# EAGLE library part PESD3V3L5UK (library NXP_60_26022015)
Low capacitance unidirectional fivefold ESD protection diode arrays Low capacitance unidirectional fivefold ElectroStatic Discharge (ESD) protection diode arrays in a leadless ultra small SOT891 Surface-Mounted Device (SMD) plastic package designed to protect up to five unidirectional signal lines from the damage caused by ESD and other transients. AAL Eindhoven MK
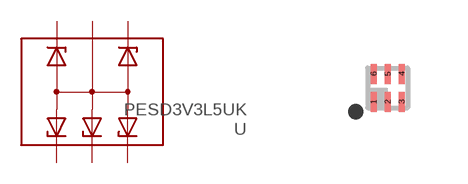
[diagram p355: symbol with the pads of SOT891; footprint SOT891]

Designator prefix U

## PESD3V3L5UK  [SOT891]
1  K1  pas
2  CA  pas
3  K2  pas
4  K3  pas
5  K4  pas
6  K5  pas

## Footprint SOT891 (pad centres in mm)
SOT891 XSON6: plastic extremely thin small outline package; no leads; 6 terminals; body 1 x 1 x 0.5 mm JEDEC: -- IEC: ---
smd 0.15 x 0.5: 1 -0.35,-0.35; 2 0,-0.35; 3 0.35,-0.35; 4 0.35,0.35; 5 0,0.35; 6 -0.35,0.35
